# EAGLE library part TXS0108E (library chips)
TXS0108E 8-Bit Bi-directional Voltage Translator
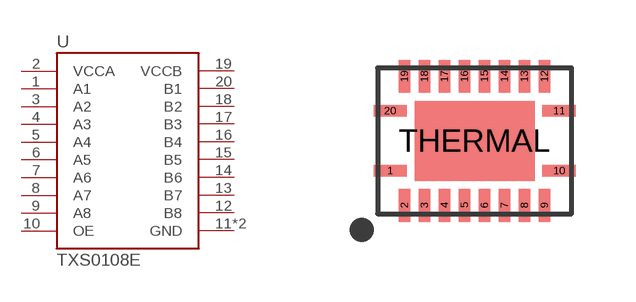
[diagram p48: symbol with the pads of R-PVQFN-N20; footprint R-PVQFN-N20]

Designator prefix U

## TXS0108EVQFN20  [R-PVQFN-N20]
1  A1
2  VCCA
3  A2
4  A3
5  A4
6  A5
7  A6
8  A7
9  A8
10  OE
11  GND
12  B8
13  B7
14  B6
15  B5
16  B4
17  B3
18  B2
19  VCCB
20  B1
THERMAL  GND

## Footprint R-PVQFN-N20 (pad centres in mm)
R-PVQFN-N20 Per TI's guidelines: http://www.ti.com/lit/an/scba017d/scba017d.pdf
smd 0.825 x 0.28: 1 -2.112,-0.75; 10 2.112,-0.75; 11 2.112,0.75; 20 -2.112,0.75
smd 0.28 x 0.825: 2 -1.75,-1.613; 3 -1.25,-1.613; 4 -0.75,-1.613; 5 -0.25,-1.613; 6 0.25,-1.613; 7 0.75,-1.613; 8 1.25,-1.613; 9 1.75,-1.613; 12 1.75,1.613; 13 1.25,1.613; 14 0.75,1.613; 15 0.25,1.613; 16 -0.25,1.613; 17 -0.75,1.613; 18 -1.25,1.613; 19 -1.75,1.613
smd 3 x 2: THERMAL 0,0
